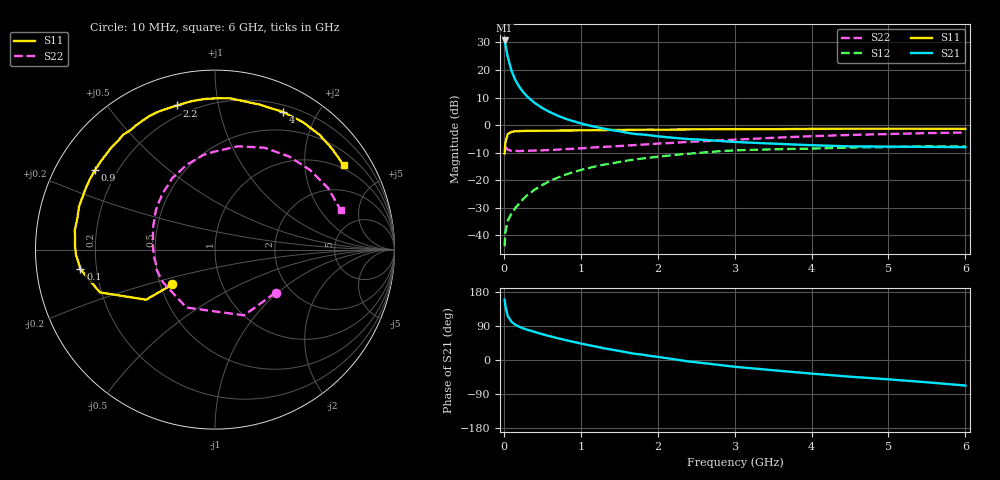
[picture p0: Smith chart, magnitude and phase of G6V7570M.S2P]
! SIEMENS Small Signal Semiconductors
! BFG193
! Si NPN RF Bipolar Junction Transistor in SOT223
! VCE = 0.75 V  IC = 70 mA
! Common Emitter S-Parameters:  August  1996
# GHz  S  MA  R  50
!  f  S11  S21  S12  S22
! GHz  MAG  ANG  MAG  ANG  MAG  ANG  MAG  ANG
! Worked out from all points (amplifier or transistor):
!   36 points, 10 MHz to 6 GHz, reference 50 ohm
!   highest |S21| = 30.7 dB at 10 MHz (marker M1)
!   |S21| within 3 dB of that: start of sweep to 30.86 MHz
!   unconditionally stable (mu >= 1): start of sweep to 22.93 MHz; 101.5 MHz to end of sweep
!   at 250 MHz: K = 1.25, MAG = 16.4 dB, |S12| = -26.8 dB
!   at 1.4 GHz: K = 1.23, MAG = 3.2 dB, |S12| = -13.9 dB
!   at 6 GHz: K = 1.08, MAG = -1.9 dB, |S12| = -7.8 dB
!   S11 on the Smith chart (normalised r, x): 10 MHz: 0.58, -0.25; 100 MHz: 0.14, -0.07; 900 MHz: 0.12, +0.30; 2.2 GHz: 0.15, +0.76; 4 GHz: 0.28, +1.58; 6 GHz: 0.88, +3.12
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0.01  0.3064 -140.7  34.3 159.4  0.0064 64.1  0.4139 -35.4
0.02  0.4747 -144.0  29.26 143.4  0.0114 57.5  0.4006 -66.1
0.05  0.6842 -159.6  17.49 116.5  0.0183 48.7  0.36 -116.3
0.1  0.7573 -171.7  9.658 100.8  0.0251 52.0  0.3421 -147.7
0.15  0.775 -177.9  6.542 92.8  0.0314 55.5  0.3437 -160.6
0.2  0.7805 178.4  4.972 87.8  0.0383 59.7  0.3384 -167.6
0.25  0.7829 174.8  3.987 83.7  0.0455 61.7  0.3422 -173.4
0.3  0.7886 172.1  3.341 80.2  0.0531 62.9  0.3424 -176.7
0.4  0.7863 167.2  2.533 74.1  0.0678 63.3  0.3471 176.6
0.5  0.7949 162.3  2.042 68.1  0.082 62.3  0.3496 171.5
0.6  0.7939 158.5  1.718 62.7  0.0977 61.1  0.3541 167.4
0.7  0.7973 154.2  1.487 57.5  0.1117 59.4  0.3603 163.6
0.9  0.8016 146.3  1.182 48.0  0.1406 54.9  0.373 155.7
1.1  0.8057 139.2  0.99 39.3  0.1667 50.3  0.3881 149.2
1.7  0.8238 119.2  0.692 16.4  0.2383 34.8  0.4355 129.5
2.2  0.8304 104.7  0.59 2.4  0.2867 21.1  0.4769 114.7
2.8  0.8436 88.8  0.518 -13.0  0.3368 5.5  0.5312 97.1
3.5  0.8454 72.8  0.462 -27.0  0.365 -12.9  0.5896 77.5
4  0.8552 63.6  0.433 -35.9  0.3758 -22.4  0.6313 64.0
4.5  0.863 55.5  0.412 -44.0  0.3933 -31.9  0.6636 51.3
5.5  0.861 40.6  0.404 -58.8  0.4146 -53.3  0.7178 28.3
6  0.8569 33.3  0.399 -67.4  0.4091 -65.5  0.734 17.5
